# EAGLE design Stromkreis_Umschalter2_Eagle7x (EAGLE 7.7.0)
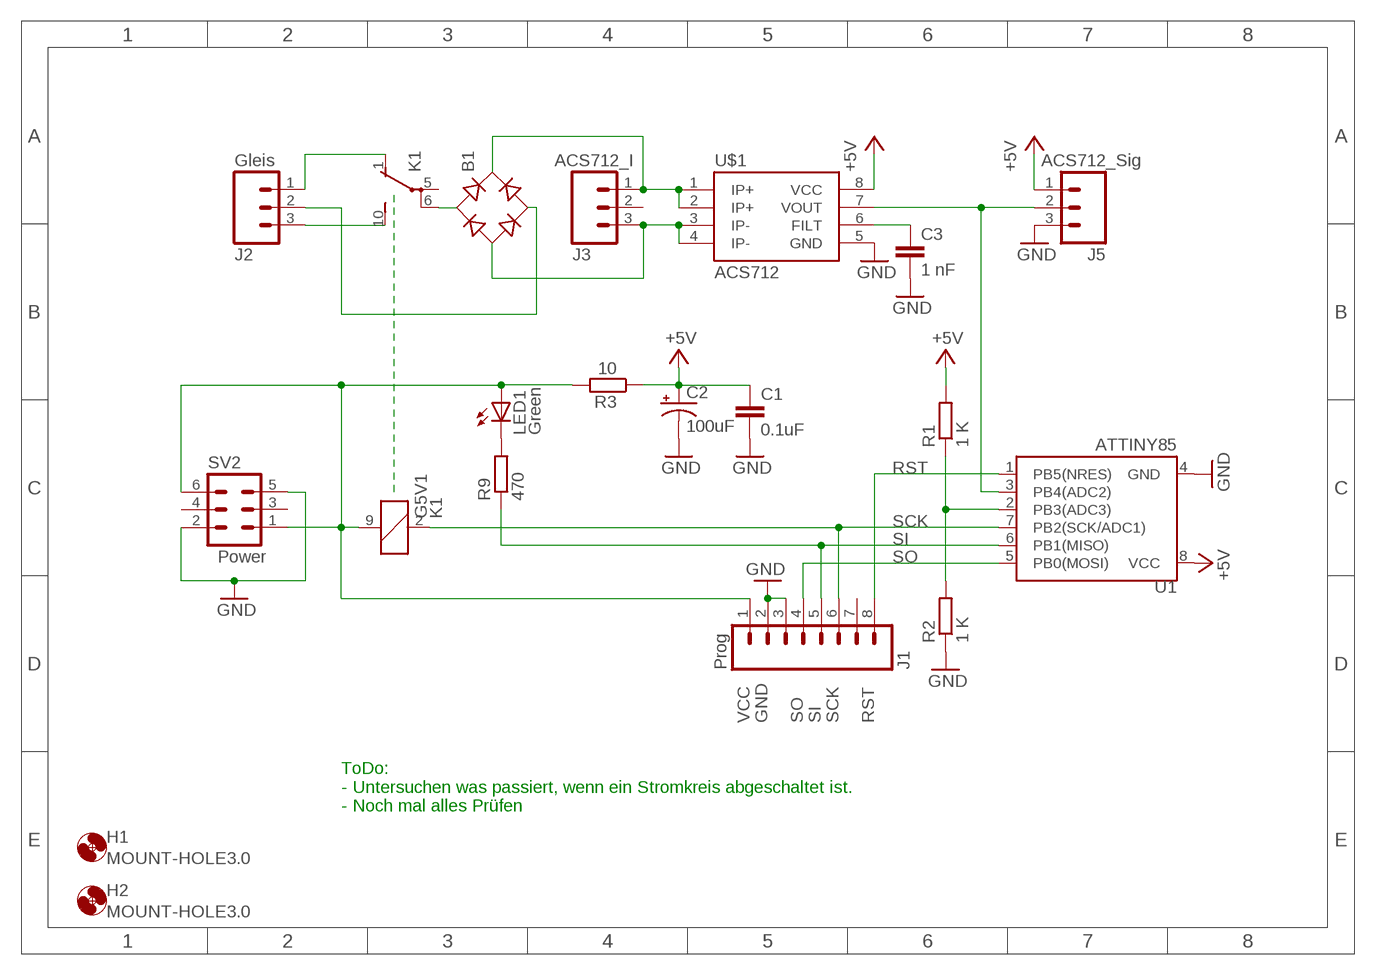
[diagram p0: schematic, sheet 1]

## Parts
B1  RB1A  [RB1A]
C1  0.1uF  0.1UF-50V-20%(PTH)KIT-EZ  [CAP-PTH-SMALL-KIT]
C2  100uF  100UF-25V-20%(PTH)  [CPOL-RADIAL-100UF-25V]
C3  1 nF  0.1UF-50V-20%(PTH)KIT-EZ  [CAP-PTH-SMALL-KIT]
H1  MOUNT-HOLE3.0  [3,0]
H2  MOUNT-HOLE3.0  [3,0]
J1  Prog  M08  [1X08_ROUND]
J2  Gleis  M03PTH  [1X03]
J3  ACS712_I  M03PTH  [1X03]
J5  ACS712_Sig  M03PTH  [1X03]
K1  G5V1  [G5V1]
LED1  Green  LED3MM  [LED3MM]
R1  1 K  R-EU_0204/7  [0204/7]
R2  1 K  R-EU_0204/7  [0204/7]
R3  10  R-EU_0204/7  [0204/7]
R9  470  R-EU_0204/7  [0204/7]
SV2  Power  ML6  [ML6]
U1  ATTINY85  ATTINY45TINY85-20-DIP  [DIP08]
U$1  ACS712  [SO08]

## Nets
+5V: C1.1 C2.1(+) J5.1 R1.2 R3.1 U1.8(VCC) U$1.8(VCC)
GND: C1.2 C2.2(-) C3.2 J1.2 J1.3 J5.3 R2.1 SV2.2 SV2.5 U1.4(GND) U$1.5(GND)
N$1: B1.AC1 K1.6(2:P)
N$2: J2.1 K1.1(2:O)
N$3: J2.3 K1.10(2:S)
N$4: B1.AC2 J2.2
N$5: B1.+ J3.1 U$1.1(IP+) U$1.2(IP+)
N$6: LED1.K(C) R9.2
N$7: C3.1 U$1.6(FILT)
N$8: J5.2 U1.3(PB4(ADC2)) U$1.7(VOUT)
N$9: R1.1 R2.2 U1.2(PB3(ADC3))
N$10: B1.- J3.3 U$1.3(IP-) U$1.4(IP-)
RST: J1.8 U1.1(PB5(NRES))
SCK: J1.6 K1.2 U1.7(PB2(SCK/ADC1))
SI: J1.5 R9.1 U1.6(PB1(MISO))
SO: J1.4 U1.5(PB0(MOSI))
VCC: J1.1 K1.9 LED1.A R3.2 SV2.1 SV2.6
Unconnected: J1.7 J3.2 K1.5(2:P) SV2.3 SV2.4

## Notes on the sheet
- ToDo:
  - Untersuchen was passiert, wenn ein Stromkreis abgeschaltet ist.
  - Noch mal alles Prüfen

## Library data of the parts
B1 = rectifier:RB1A: RECTIFIER 1 A
C1 C3 = SparkFun-Capacitors:0.1UF-50V-20%(PTH): CAP-08370; PROD_ID: CAP-08370
C2 = SparkFun-Capacitors:100UF-25V-20%(PTH): CAP-08439; PROD_ID: CAP-08439
H1 H2 = holes:MOUNT-HOLE: MOUNTING HOLE with drill center marker
J1 = SparkFun-Connectors:M08: Header 8 Standard 8-pin 0.1" header. Use with straight break away headers (SKU : PRT-00116), right angle break away headers (PRT-00553), swiss pins (PRT-00743), machine pins (PRT-00117), and female headers (PRT-00115).; PROD_ID: CONN-08437
J2 J3 J5 = SparkFun-Connectors:M03: Header 3 Standard 3-pin 0.1" header. Use with straight break away headers (SKU : PRT-00116), right angle break away headers (PRT-00553), swiss pins (PRT-00743), machine pins (PRT-00117), and female headers (PRT-00115). Molex polarized connector foot print use with SKU : PRT-08232 with associated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
K1 = relay:G5V1: RELAY 1 x switch, 0.5 A/125 V AC, 1 A/24 V DC , Omron; MPN: G5V-1-DC24; OC_FARNELL: 9949593; OC_NEWARK: 36M6377
LED1 = led:LED: LED
R1-R3 R9 = rcl:R-EU_: RESISTOR, European symbol
SV2 = con-harting-ml:ML6: HARTING; OC_FARNELL: unknown; OC_NEWARK: unknown
U1 = SparkFun-DigitalIC:ATTINY45: Atmel 8-pin 2/4/8kB flash uC; PROD_ID: IC-09445; VALUE: TINY85-20-DIP
U$1 = SparkFun-AnalogIC:ACS712: Hall-effect-based isolated linear current sensor; PROD_ID: IC-08964

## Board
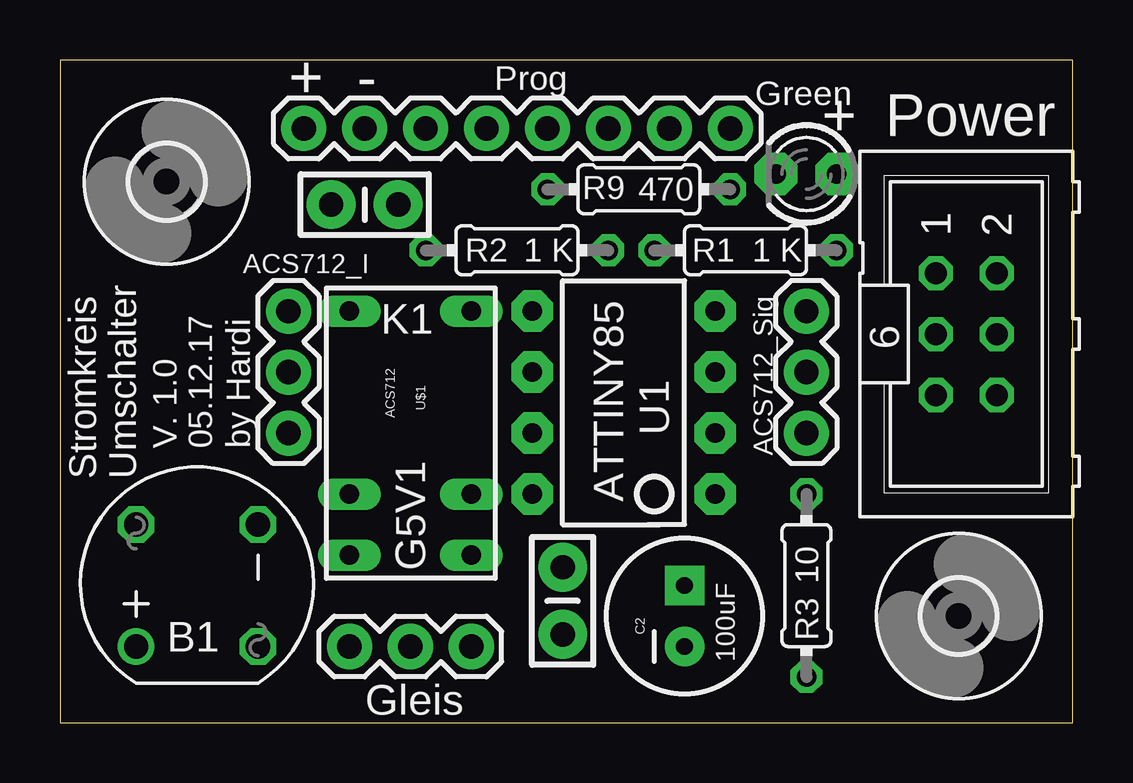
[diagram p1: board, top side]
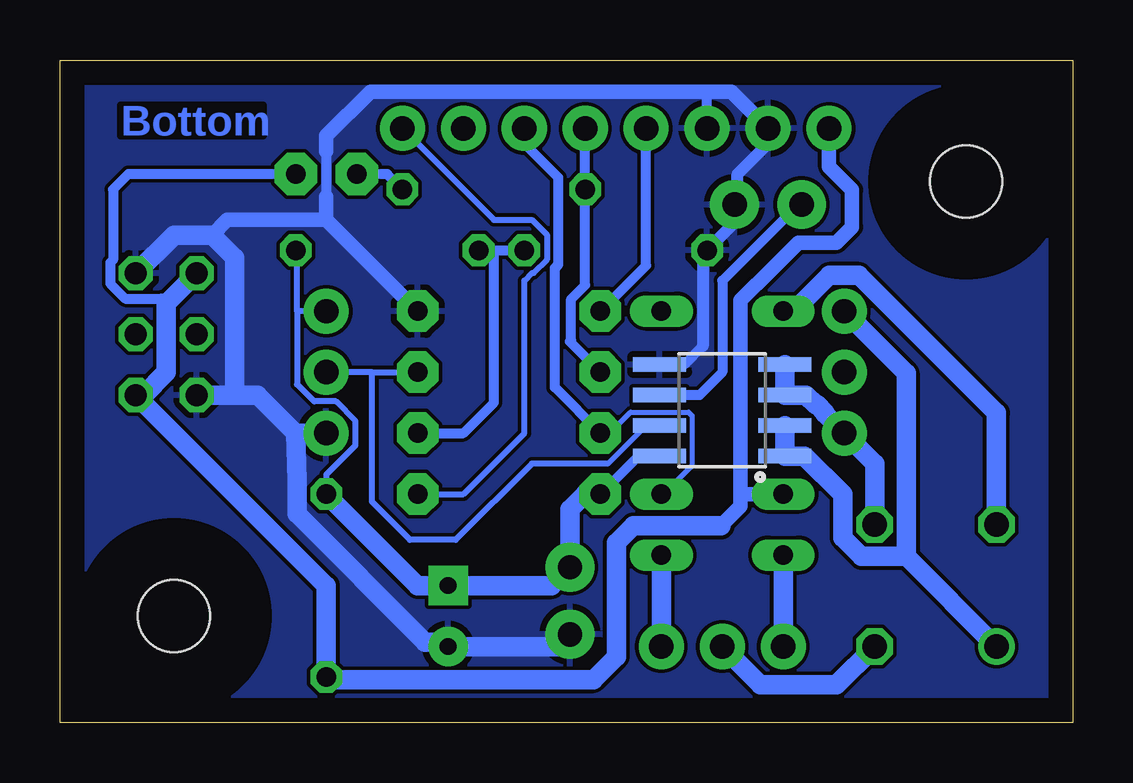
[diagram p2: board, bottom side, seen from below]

Size 42.22 x 27.61 mm. Coordinates in mm from the lower left corner, seen from the top.
Outline: 0,0 42.22,0 42.22,27.61 0,27.61 0,0
Copper layers (1*16): Top 0.035mm / dielectric 1.5mm / Bottom 0.035mm
Design rules "default": minimum track width 6mil, minimum drill 0.35mm, track to track 6mil, track to pad 6mil, pad to pad 6mil, via to via 6mil, smd to smd 6mil, copper to edge 40mil, drill to drill 6mil, minimum pad ring 10mil, minimum via ring 8mil, stop-mask expansion 4mil, vias tented up to drill 0mil, thermal gap 10mil

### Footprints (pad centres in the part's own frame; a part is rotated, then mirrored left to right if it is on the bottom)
RB1A = drill 1.016: + -2.54,2.54 | drill 1.016 octagon: - 2.54,-2.54; AC1 2.54,2.54; AC2 -2.54,-2.54
CAP-PTH-SMALL-KIT = drill 1.016 pad 2.032: 1 -1.397,0; 2 1.397,0
CPOL-RADIAL-100UF-25V = drill 0.7 pad 1.651 square: 1 1.27,0 | drill 0.7 pad 1.651: 2 -1.27,0
3,0 = hole 3: 0,0
1X08_ROUND = drill 1.016 pad 1.88: 1 0,0; 2 2.54,0; 3 5.08,0; 4 7.62,0; 5 10.16,0; 6 12.7,0; 7 15.24,0; 8 17.78,0
1X03 = drill 1.016 pad 1.88: 1 0,0; 2 2.54,0; 3 5.08,0
G5V1 = drill 0.813 long: 1 -5.08,-2.54; 2 -2.54,-2.54; 5 5.08,-2.54; 6 5.08,2.54; 9 -2.54,2.54; 10 -5.08,2.54
LED3MM = drill 0.813 pad 1.778 octagon: A -1.27,0; K 1.27,0
0204/7 = drill 0.813 octagon: 1 -3.81,0; 2 3.81,0
ML6 = drill 0.914 octagon: 1 -2.54,-1.27; 2 -2.54,1.27; 3 0,-1.27; 4 0,1.27; 5 2.54,-1.27; 6 2.54,1.27
DIP08 = drill 0.813 pad 1.727 octagon: 1 -3.81,-3.81; 2 -1.27,-3.81; 3 1.27,-3.81; 4 3.81,-3.81; 5 3.81,3.81; 6 1.27,3.81; 7 -1.27,3.81; 8 -3.81,3.81
SO08 = smd 0.61 x 2.21: 1 -1.905,-2.616; 2 -0.635,-2.616; 3 0.635,-2.616; 4 1.905,-2.616; 5 1.905,2.616; 6 0.635,2.616; 7 -0.635,2.616; 8 -1.905,2.616

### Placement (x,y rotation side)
B1  5.71,5.71 90 top
C1  20.95,5.08 270 top
C2  26.04,4.45 90 top
C3  12.7,21.59 0 top
H1  37.47,4.45 0 top
H2  4.45,22.54 0 top
J1  10.16,24.77 0 top
J2  17.14,3.17 180 top
J3  9.53,17.14 270 top
J5  31.11,17.14 270 top
K1  14.61,12.06 90 top
LED1  31.11,22.86 180 top
R1  28.57,19.68 0 top
R2  19.05,19.68 0 top
R3  31.11,5.71 270 top
R9  24.13,22.23 0 top
SV2  37.78,16.19 270 top
U1  23.49,13.34 90 top
U$1  14.61,13.02 90 bottom

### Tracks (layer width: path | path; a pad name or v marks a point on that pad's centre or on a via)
+5V
  Bottom 0.254: R3.1 31.11,10.34 29.9,11.56 29.9,12.57 30.71,13.39 31.62,13.39 32.33,14.1 32.33,17.14 | R1.2 32.33,19.63 32.33,17.14 | J5.1 32.33,17.14
  Bottom 0.406: U$1.8 18.1,11.11 U1.8
  Bottom 0.813: 25.91,5.84 C2.1 | U1.8 20.32,9.53 20.95,8.89 C1.1 21.72,5.71 C2.1 | C2.1 27.3,5.71 R3.1
GND
  Bottom 0.406: 15.42,15.7 16.19,14.92 U$1.5 | 31.11,23.81 31.11,21.91 | J1.3 15.24,26.29
  Bottom 0.508: 15.42,15.7 15.42,19.51 R2.1 14.1,20.83 C3.2 13.97,21.72 13.97,22.86 12.7,24.13 J1.2
  Bottom 0.61: 31.11,20.95 35.24,20.95 35.88,20.32 | J1.2 14.23,26.29 15.24,26.29 29.27,26.29 31.11,24.45 31.11,23.81 | 31.11,21.91 31.11,20.95 | 31.11,20.95 U1.4
  Bottom 0.813: C1.2 21.46,3.17 C2.2 26.22,3.36 26.99,3.36 32.33,8.7 32.33,10.11 32.39,12.06 | J5.3 32.39,12.06 | 32.39,12.06 33.97,13.65 34.93,13.65 | 34.93,13.65 SV2.5 | 34.93,13.65 34.93,19.37 35.88,20.32 37.47,20.32 SV2.2
  pour Bottom: 0.32,0.32 41.91,0.32 41.91,27.3 0.32,27.3
N$1
  Bottom 0.813: K1.6 11.64,17.14 10.15,18.64 8.9,18.64 3.17,12.91 B1.AC1
N$2
  Bottom 0.813: J2.1 K1.1
N$3
  Bottom 0.813: J2.3 K1.10
N$4
  Bottom 0.813: B1.AC2 9.84,1.59 13.02,1.59 J2.2
N$5
  Bottom 0.61: 6.93,6.93 7.04,7.04
  Bottom 0.813: 6.93,6.93 B1.+ | 6.93,6.93 8.8,6.93 9.58,7.71 9.58,9.51 11.18,11.11 U$1.1 U$1.2 | J3.1 6.93,14.55 6.93,6.93
N$6
  Bottom 0.406: R9.2 28.57,22.86 LED1.K
N$7
  Bottom 0.406: C3.1 11.43,21.59 14.61,18.41 14.61,14.61 15.56,13.65 U$1.6
N$8
  Bottom 0.203: U$1.7 17.79,12.38 19.21,10.96 | 19.21,10.96 19.22,10.95 | 19.21,10.96 19.37,10.79
  Bottom 0.254: 29.21,14.61 U1.3 | 29.21,14.61 J5.2 | 19.37,10.79 22.54,10.79 25.72,7.62 27.62,7.62 29.21,9.21 29.21,14.61
N$9
  Bottom 0.406: U1.2 25.4,12.06 24.13,13.34 24.13,19.68 | 24.13,19.68 R1.1 | 24.13,19.68 R2.2
N$10
  Bottom 0.813: B1.- 8.26,10.79 J3.3 10.33,12.87 10.33,12.92 10.65,13.25 10.71,13.25 11.11,13.65 U$1.3 U$1.4
RST
  Bottom 0.254: J1.8 24.13,20.95 22.54,20.95 21.92,20.33 21.92,19.3 22.47,18.75 22.53,18.75 22.86,18.41 22.86,12.06 25.4,9.53 U1.1
SCK
  Bottom 0.203: U1.7 19.31,12.06 18.43,12.94 16.01,12.94 15.86,12.79 15.86,10.7 16.51,10.05 16.51,9.84 16.83,9.53 K1.2
  Bottom 0.406: U1.7 21.59,13.97 21.59,18.94 21.44,19.1 21.44,22.71 22.86,24.13 J1.6
SI
  Bottom 0.406: U1.6 20.95,15.88 20.9,15.93 20.9,17.65 20.32,18.23 R9.1 J1.5
SO
  Bottom 0.406: U1.5 17.78,19.05 J1.4
VCC
  Bottom 0.406: LED1.A 39.37,22.86 40.01,22.23 40.01,19.29 40.12,19.17 40.12,18.29 39.49,17.67 37.99,17.67 37.78,17.46
  Bottom 0.61: J1.1 10.16,23.16 9.2,22.2 9.2,20.65 9.84,20 11.43,20 13.17,18.26 13.19,18.26 13.84,17.61 13.84,9.53 | 14.66,8.2 13.84,9.02 13.84,9.53 | K1.9 13.84,9.53
  Bottom 0.813: 14.66,8.2 18.31,8.2 19.02,7.49 19.02,2.75 19.98,1.79 31.1,1.79 31.1,1.89 R3.2 31.11,5.71 SV2.6 38.73,13.65 37.78,14.61 37.78,17.46 SV2.1

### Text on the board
Bottom: Bottom
tNames: + | - | + | V. 1.0 / 05.12.17 | by Hardi | Stromkreis / Umschalter

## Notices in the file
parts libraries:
SparkFun-AnalogIC: Licensing:Creative Commons ShareAlike 4.0 International - https://creativecommons.org/licenses/by-sa/4.0
